(* Logix 5000 Rung export; software revision 16.03 *)

MODULES
   Local : vendor None type None code None
   GSC : vendor None type None code None
END_MODULES

TYPE GSCMODULEDEF :   // This define the complete module tags
STRUCT
   CONFIG : GSCPORTCONFIG;   // Port configuration parameters
   DATA : GSCDATA;   // Port sent and received data
   STATUS : GSCSTATUS;   // Module status data and individual port status
   CONTROL : GSCCONTROL;   // Module control parameters
   UTIL : GSCUTIL;   // Tags used by the module
END_STRUCT
END_TYPE

TYPE GSCPORTCONFIG :   // Shows both ports configuration
STRUCT
   Port1 : GSCPORTCONFIGPARA;   // Port 1 configuration data
   Port2 : GSCPORTCONFIGPARA;   // Port 2 configuration data
END_STRUCT
END_TYPE

TYPE GSCPORTSTAT :   // Port status Data
STRUCT
   RxState : INT;   // State of receive task
   RxCharCnt : INT;   // Number of characters received on port
   RxMsgCnt : INT;   // Number of messages received on port
   TxState : INT;   // State of transmit task
   TxCharCnt : INT;   // Number of characters transmitted on port
   TxMsgCnt : INT;   // Number of messages transmitted on port
   ErrorWord : GSCERRORWORD;   // Error/Configuration Word for port
END_STRUCT
END_TYPE

TYPE GSCCONTROL :   // Ladder send special blocks to request the module to perform the request
STRUCT
   Warmboot : BOOL;   // Performs a warm boot operation on the module (software reset).
   Coldboot : BOOL;   // Performs a cold boot operation on the module (hardware and software reset).
   ConfigDone : BOOL;   // This to confirm the module reveived its configuration from ladder logic
END_STRUCT
END_TYPE

TYPE GSCPORTCONFIGPARA :   // The following are the configuration parameters for the port of the MVI56-GSC module.
STRUCT
   Enabled : INT;   // 0=Disable port, 1=Enable port
   Type : INT;   // Type of control used to flush data received on port
   Baudrate : INT;   // Baud rate for communications
   Parity : INT;   // Parity (0=none, 1=odd, 2=even, 3=mark, 4=space)
   DataBits : INT;   // Data bits (5, 6, 7, or 8)
   StopBits : INT;   // Stop bits (1 or 2)
   RTSOn : INT;   // RTS delay before sending data
   RTSOff : INT;   // RTS delay after sending message
   Handshaking : INT;   // Type of Handshaking (0=none, 1=RTSCTS, 2=DTRDSR,3=XONXOFF)
   RTermCnt : INT;   // Number of termination characters for received message for control
   RTermChar : SINT[12];   // Characters for termination control
   RPacketLen : INT;   // Fixed packet length value
   RTimeout : INT;   // Message timeout value for control
   RDelay : INT;   // Intercharacter timeout for control
   WTermCnt : INT;   // Not used
   WTermChar : SINT[12];   // Not used
   WPacketLen : INT;   // Not used
   WTimeout : INT;   // Timeout for sending a message out the port
   Spare : INT;   // Not used
   WMinDelay : INT;   // Minimum delay before transmitting message out port
END_STRUCT
END_TYPE

TYPE GSCBLOCKSTATUS :   // This shows all blocks that were used by the module
STRUCT
   Read : INT;   // Number of blocks read by the module
   Write : INT;   // Number of blocks written by the module
   Parse : INT;   // Number of blocks parsed by the module
   Err : INT;   // Number of block transfer errors
END_STRUCT
END_TYPE

TYPE GSCERRORWORD :   // Bit coded error word for configuration and overflow error for MVI56-GSC module.
STRUCT
   Cfg_type : BOOL;   // Bit 0, type field configuration error
   Cfg_Baud : BOOL;   // Bit 1, baud rate field configuration error
   Cfg_Parity : BOOL;   // Bit 2, parity field configuration error
   Cfg_DataBits : BOOL;   // Bit 3, data bit field configuration error
   Cfg_StopBits : BOOL;   // Bit 4, stop bit field configuration error
   Cfg_Handshake : BOOL;   // Bit 5, handshaking field configuration error
   Cfg_RTermcount : BOOL;   // Bit 6, receive termination character count field configuration error
   Cfg_RPacketLen : BOOL;   // Bit 7, receive packet length field configuration error
   Cfg_RTimeout : BOOL;   // Bit 8, receive message timeout field configuration error
   Cfg_RDelay : BOOL;   // Bit 9, receive intercharacter delay field configuration error
   Cfg_WTimeout : BOOL;   // Bit 10, write message timeout field configuration error
   Resv_Bit11 : BOOL;   // Bit 11
   Resv_Bit12 : BOOL;   // Bit 12
   Resv_Bit13 : BOOL;   // Bit 13
   Resv_Bit14 : BOOL;   // Bit 14
   Err_ROverflow : BOOL;   // Bit 15, receive overflow error
END_STRUCT
END_TYPE

TYPE GSCPORTDATA :   // Individual port data
STRUCT
   ReadLength : INT;   // The length of character the port is rescieving
   ReadString : SINT[4096];   // Where received data will be displayed
   WriteLength : INT;   // The length of character the port is transmitting
   WDelay : INT;   // Number of milliseconds to wait between each character sent from the port
   WriteString : SINT[4096];   // Where sent data will be placed before it is sent
END_STRUCT
END_TYPE

TYPE GSCDATA :   // The following contains the data read in on the port and to be written out the port.
STRUCT
   Port1 : GSCPORTDATA;   // Port 1 data
   Port2 : GSCPORTDATA;   // Port 2 data
END_STRUCT
END_TYPE

TYPE GSCUTIL :   // Used by the module for block hand shaking
STRUCT
   LastRead : SINT;   // This is used to read the input image from the processor
   LastWrite : SINT;   // This is used to write the output image to the processor
   BackplaneFail : INT;   // This is used to control number of backplane failures before module stops communicating on both gsc ports
   P1WriteLast : INT;   // Port 1 last write data in the array
   P2Writelast : INT;   // Port 2 last data in the array
   P1ArrayIndex : INT;   // This is the index reference within the read or write data array for port1
   P2ArrayIndex : INT;   // This is the index reference within the read or write data array for port 2
   P1RSindex : INT;   // used when more than 200 characters are received on the port 1
   P2RSindex : INT;   // used when more than 200 characters are received on the port 2
   P1Temp1 : INT;   // This temp parameter for port 1 is used to copy SINT to and INT in order to read a vlaue is higher than 127 characheters
   P2Temp2 : INT;   // This temp parameter for port 2 is used to copy SINT to and INT in order to read a vlaue is higher than 127 characheters
   Scratch1 : INT;   // Used to calculate number of characters read by the port
   Scratch2 : INT;   // Used to calculate number of characters read by the port
END_STRUCT
END_TYPE

TYPE GSCSTATUS :   // Module Status data
STRUCT
   PassCnt : INT;   // Program cycle counter for module
   Product : INT[2];   // Product code for module (GSC)
   Rev : INT[2];   // Revision level of module's code
   OP : INT[2];   // Operating system version for module
   Run : INT[2];   // Run number for module
   BlockStatus : GSCBLOCKSTATUS;   // Data block transfer statistics
   Port1 : GSCPORTSTAT;   // Status for port1
   Port2 : GSCPORTSTAT;   // Status for port 2
END_STRUCT
END_TYPE

ADD_ON_INSTRUCTION AOI56GSC   (* revision 1.7, vendor ProSoft Technology Inc., ExecutePrescan *)
// Add-On For MVI56GSC and MVI56EGSC Modules.
// Revision note:
// 05/09/13
// AOI was fixed so that GSC.UTIL.Backplane.Fail parameter was affecting the intercharacter delay parameter in the module
VAR_IN_OUT
   Connection_Input : SINT[500]; {required}
   Connection_Output : SINT[496]; {required}
   GSC : GSCMODULEDEF; {required}
END_VAR
VAR
   MJFAULTS : DINT[12];
   ONS_Config : BOOL;
END_VAR

ROUTINE Logic   (* ladder *)
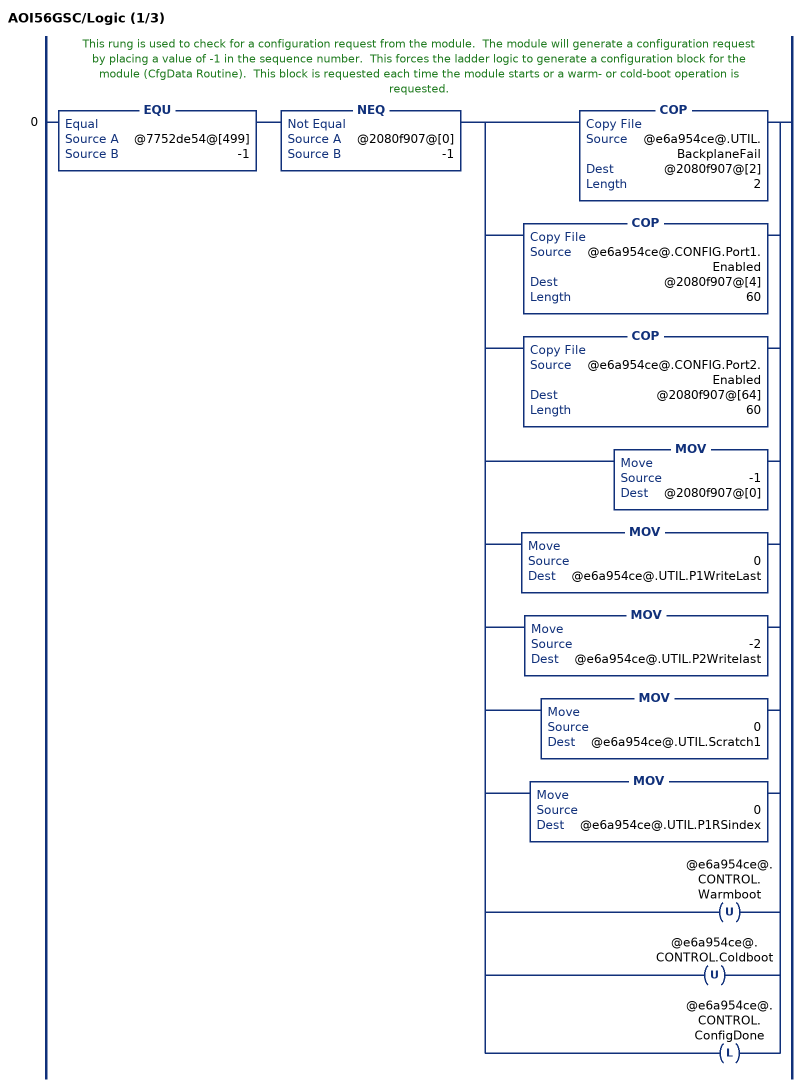
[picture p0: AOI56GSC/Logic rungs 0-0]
   // This rung is used to check for a configuration request from the module.  The module will generate a configuration request by placing a value of -1 in the sequence number.  This forces the ladder logic to generate a configuration block for the module (CfgData Routine).  This block is requested each time the module starts or a warm- or cold-boot operation is requested.
   0: EQU(@7752de54@[499],-1)NEQ(@2080f907@[0],-1)[COP(@e6a954ce@.UTIL.BackplaneFail,@2080f907@[2],2) ,COP(@e6a954ce@.CONFIG.Port1.Enabled,@2080f907@[4],60) ,COP(@e6a954ce@.CONFIG.Port2.Enabled,@2080f907@[64],60) ,MOV(-1,@2080f907@[0]) ,MOV(0,@e6a954ce@.UTIL.P1WriteLast) ,MOV(-2,@e6a954ce@.UTIL.P2Writelast) ,MOV(0,@e6a954ce@.UTIL.Scratch1) ,MOV(0,@e6a954ce@.UTIL.P1RSindex) ,OTU(@e6a954ce@.CONTROL.Warmboot) ,OTU(@e6a954ce@.CONTROL.Coldboot) ,OTL(@e6a954ce@.CONTROL.ConfigDone) ];
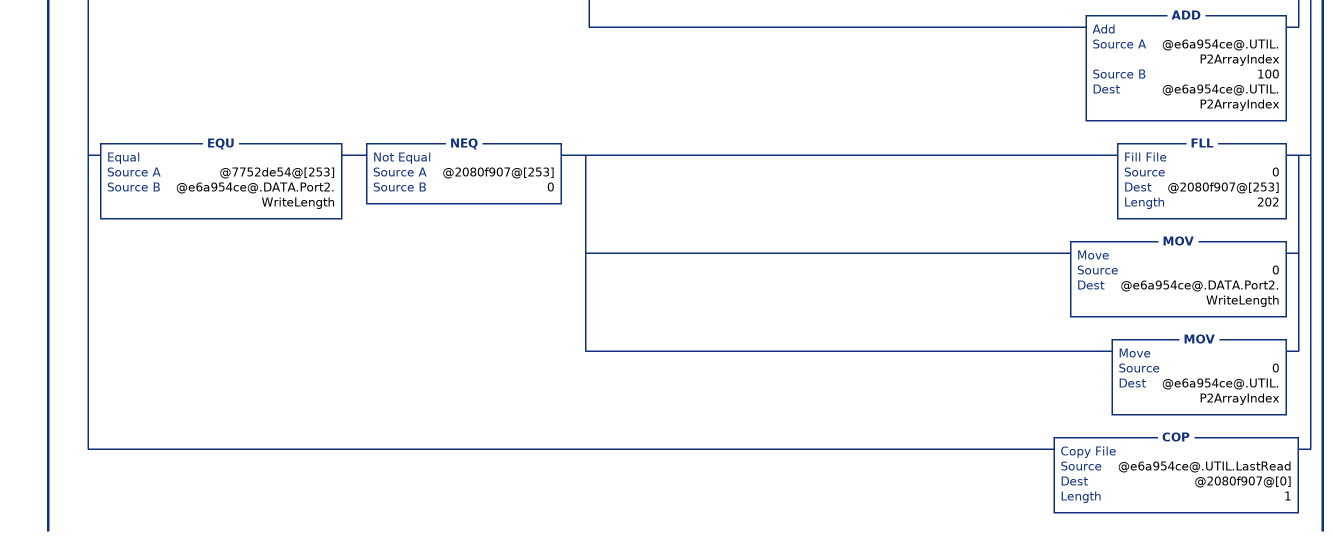
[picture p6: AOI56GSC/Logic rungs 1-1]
   // This rung is executed when a new data block is received from the module.  These blocks will have a sequence number range of 0 to 127.  When a new block is received, the ProcessBlock routine is executed to handle the newly received data.
   1: NEQ(@7752de54@[499],@e6a954ce@.UTIL.LastRead)NEQ(@7752de54@[499],-1)XIO(@e6a954ce@.CONTROL.Warmboot)XIO(@e6a954ce@.CONTROL.Coldboot)[COP(@7752de54@[499],@e6a954ce@.UTIL.LastRead,1) ,GEQ(@e6a954ce@.UTIL.LastRead,0) [COP(@7752de54@[210],@e6a954ce@.STATUS.PassCnt,1) ,COP(@7752de54@[1],@e6a954ce@.UTIL.P1Temp1,1) ,COP(@7752de54@[251],@e6a954ce@.UTIL.P2Temp2,1) ,COP(@7752de54@[212],@e6a954ce@.STATUS.Product[0],8) ,COP(@7752de54@[228],@e6a954ce@.STATUS.BlockStatus.Read,4) ,COP(@7752de54@[236],@e6a954ce@.STATUS.Port1.RxState,6) ,COP(@7752de54@[248],@e6a954ce@.STATUS.Port1.ErrorWord,1) ,COP(@7752de54@[456],@e6a954ce@.STATUS.Port2.RxState,6) ,COP(@7752de54@[468],@e6a954ce@.STATUS.Port2.ErrorWord,1) ,EQU(@e6a954ce@.UTIL.P1Temp1,-1) LES(@e6a954ce@.UTIL.P1RSindex,20) [COP(@7752de54@[5],@e6a954ce@.DATA.Port1.ReadString[@e6a954ce@.UTIL.P1RSindex*200],200) ,ADD(1,@e6a954ce@.UTIL.P1RSindex,@e6a954ce@.UTIL.P1RSindex) ,MUL(@e6a954ce@.UTIL.P1RSindex,200,@e6a954ce@.UTIL.Scratch1) ] ,GRT(@e6a954ce@.UTIL.P1Temp1,0) [MOV(0,@e6a954ce@.DATA.Port1.ReadLength) ,COP(@7752de54@[5],@e6a954ce@.DATA.Port1.ReadString[@e6a954ce@.UTIL.P1RSindex*200],200) ,ADD(@e6a954ce@.UTIL.P1Temp1,@e6a954ce@.UTIL.Scratch1,@e6a954ce@.DATA.Port1.ReadLength) ,MOV(0,@e6a954ce@.UTIL.P1RSindex) ,MOV(0,@e6a954ce@.UTIL.Scratch1) ] ,EQU(@e6a954ce@.UTIL.P2Temp2,-1) LES(@e6a954ce@.UTIL.P2RSindex,20) [COP(@7752de54@[255],@e6a954ce@.DATA.Port2.ReadString[@e6a954ce@.UTIL.P2RSindex*200],200) ,ADD(1,@e6a954ce@.UTIL.P2RSindex,@e6a954ce@.UTIL.P2RSindex) ,MUL(@e6a954ce@.UTIL.P2RSindex,200,@e6a954ce@.UTIL.Scratch2) ] ,GRT(@e6a954ce@.UTIL.P2Temp2,0) [MOV(0,@e6a954ce@.DATA.Port2.ReadLength) ,COP(@7752de54@[255],@e6a954ce@.DATA.Port2.ReadString[@e6a954ce@.UTIL.P2RSindex*200],200) ,ADD(@e6a954ce@.UTIL.P2Temp2,@e6a954ce@.UTIL.Scratch2,@e6a954ce@.DATA.Port2.ReadLength) ,MOV(0,@e6a954ce@.UTIL.P2RSindex) ,MOV(0,@e6a954ce@.UTIL.Scratch2) ] ] ,XIC(@e6a954ce@.CONTROL.ConfigDone) [FLL(0,@2080f907@[1],496) ,OTU(@e6a954ce@.CONTROL.ConfigDone) ] ,GRT(@e6a954ce@.DATA.Port1.WriteLength,100) LEQ(@e6a954ce@.DATA.Port1.WriteLength,4096) [COP(@e6a954ce@.DATA.Port1.WriteString[@e6a954ce@.UTIL.P1ArrayIndex],@2080f907@[5],100) ,MOV(100,@2080f907@[3]) ] ,GRT(@e6a954ce@.DATA.Port1.WriteLength,0) LEQ(@e6a954ce@.DATA.Port1.WriteLength,100) [COP(@e6a954ce@.DATA.Port1.WriteString[@e6a954ce@.UTIL.P1ArrayIndex],@2080f907@[5],@e6a954ce@.DATA.Port1.WriteLength) ,COP(@e6a954ce@.DATA.Port1.WDelay,@2080f907@[1],2) ,MOV(@e6a954ce@.DATA.Port1.WriteLength,@2080f907@[3]) ] ,NEQ(@7752de54@[3],@e6a954ce@.DATA.Port1.WriteLength) GRT(@7752de54@[3],0) [FLL(0,@2080f907@[3],202) ,SUB(@e6a954ce@.DATA.Port1.WriteLength,100,@e6a954ce@.DATA.Port1.WriteLength) ,ADD(@e6a954ce@.UTIL.P1ArrayIndex,100,@e6a954ce@.UTIL.P1ArrayIndex) ] ,EQU(@7752de54@[3],@e6a954ce@.DATA.Port1.WriteLength) NEQ(@2080f907@[3],0) [FLL(0,@2080f907@[3],202) ,MOV(0,@e6a954ce@.DATA.Port1.WriteLength) ,MOV(0,@e6a954ce@.UTIL.P1ArrayIndex) ] ,GRT(@e6a954ce@.DATA.Port2.WriteLength,100) LEQ(@e6a954ce@.DATA.Port2.WriteLength,4096) [COP(@e6a954ce@.DATA.Port2.WriteString[@e6a954ce@.UTIL.P2ArrayIndex],@2080f907@[255],100) ,MOV(100,@2080f907@[253]) ] ,GRT(@e6a954ce@.DATA.Port2.WriteLength,0) LEQ(@e6a954ce@.DATA.Port2.WriteLength,100) [COP(@e6a954ce@.DATA.Port2.WriteString[@e6a954ce@.UTIL.P2ArrayIndex],@2080f907@[255],@e6a954ce@.DATA.Port2.WriteLength) ,COP(@e6a954ce@.DATA.Port2.WDelay,@2080f907@[251],2) ,MOV(@e6a954ce@.DATA.Port2.WriteLength,@2080f907@[253]) ] ,NEQ(@7752de54@[253],@e6a954ce@.DATA.Port2.WriteLength) GRT(@7752de54@[253],0) [FLL(0,@2080f907@[253],202) ,SUB(@e6a954ce@.DATA.Port2.WriteLength,100,@e6a954ce@.DATA.Port2.WriteLength) ,ADD(@e6a954ce@.UTIL.P2ArrayIndex,100,@e6a954ce@.UTIL.P2ArrayIndex) ] ,EQU(@7752de54@[253],@e6a954ce@.DATA.Port2.WriteLength) NEQ(@2080f907@[253],0) [FLL(0,@2080f907@[253],202) ,MOV(0,@e6a954ce@.DATA.Port2.WriteLength) ,MOV(0,@e6a954ce@.UTIL.P2ArrayIndex) ] ,COP(@e6a954ce@.UTIL.LastRead,@2080f907@[0],1) ];
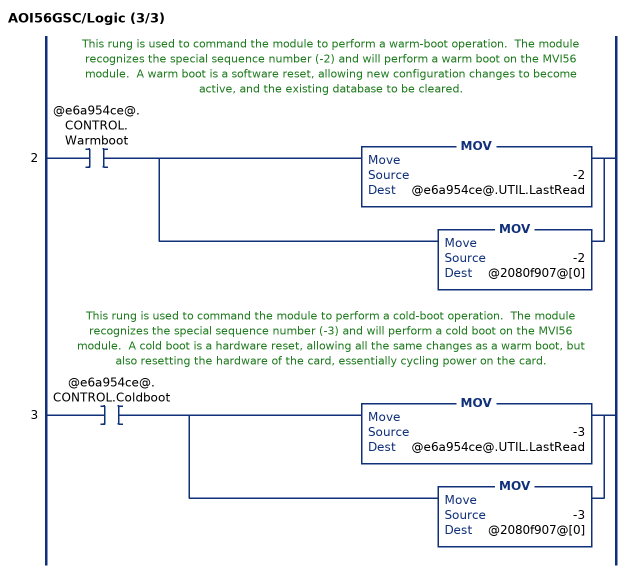
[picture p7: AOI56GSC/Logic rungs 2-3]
   // This rung is used to command the module to perform a warm-boot operation.  The module recognizes the special sequence number (-2) and will perform a warm boot on the MVI56 module.  A warm boot is a software reset, allowing new configuration changes to become active, and the existing database to be cleared.
   2: XIC(@e6a954ce@.CONTROL.Warmboot)[MOV(-2,@e6a954ce@.UTIL.LastRead) ,MOV(-2,@2080f907@[0]) ];
   // This rung is used to command the module to perform a cold-boot operation.  The module recognizes the special sequence number (-3) and will perform a cold boot on the MVI56 module.  A cold boot is a hardware reset, allowing all the same changes as a warm boot, but also resetting the hardware of the card, essentially cycling power on the card.
   3: XIC(@e6a954ce@.CONTROL.Coldboot)[MOV(-3,@e6a954ce@.UTIL.LastRead) ,MOV(-3,@2080f907@[0]) ];
END_ROUTINE

ROUTINE Prescan   (* ladder *)
// PowerUp
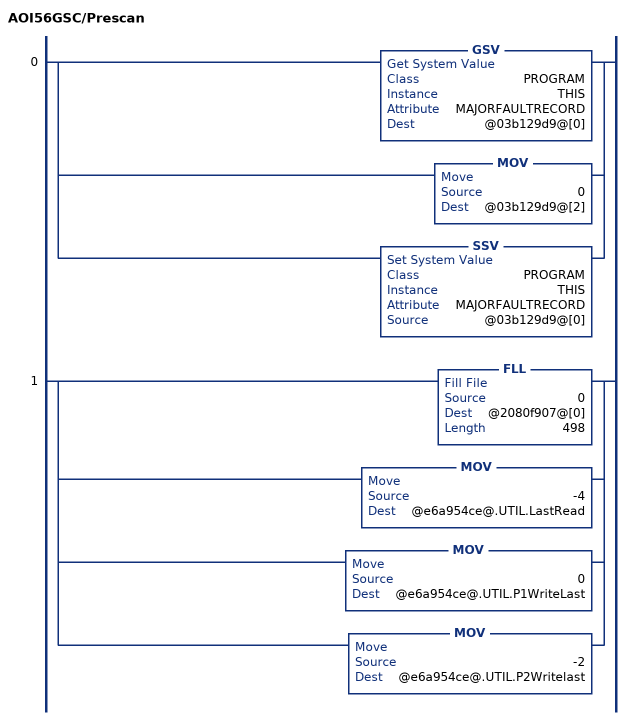
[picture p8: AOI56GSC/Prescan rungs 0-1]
   0: [GSV(PROGRAM,THIS,MAJORFAULTRECORD,@03b129d9@[0]) ,MOV(0,@03b129d9@[2]) ,SSV(PROGRAM,THIS,MAJORFAULTRECORD,@03b129d9@[0]) ];
   1: [FLL(0,@2080f907@[0],498) ,MOV(-4,@e6a954ce@.UTIL.LastRead) ,MOV(0,@e6a954ce@.UTIL.P1WriteLast) ,MOV(-2,@e6a954ce@.UTIL.P2Writelast) ];
END_ROUTINE
END_ADD_ON_INSTRUCTION

VAR_GLOBAL   (* controller tags *)
   Local:1:I : AB:1756_MODULE_SINT_500Bytes:I:0;
   AOI56GSC : AOI56GSC;
   GSC : GSCMODULEDEF;
   Local:1:O : AB:1756_MODULE_SINT_496Bytes:O:0;
END_VAR

PROGRAM MainProgram

ROUTINE MainRoutine   (* ladder *)
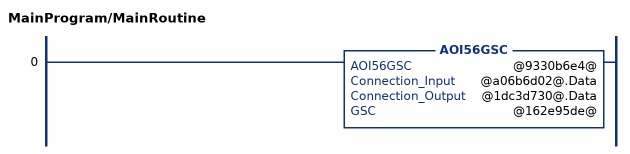
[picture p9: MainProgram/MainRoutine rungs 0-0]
   0: AOI56GSC(@9330b6e4@,@a06b6d02@.Data,@1dc3d730@.Data,@162e95de@);
END_ROUTINE
END_PROGRAM
